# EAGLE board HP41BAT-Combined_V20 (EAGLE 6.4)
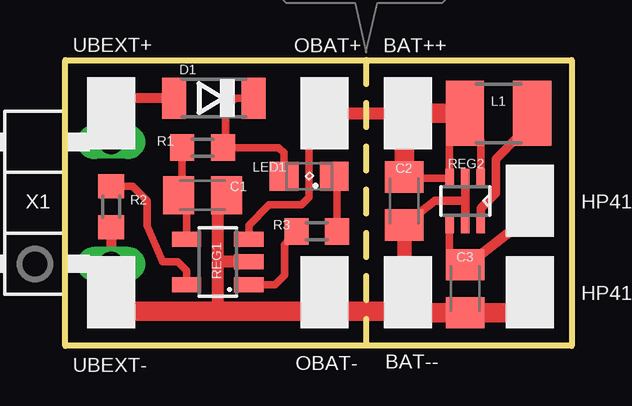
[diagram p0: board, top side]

Size 21.11 x 11.91 mm. Coordinates in mm from the lower left corner, seen from the top.
Outline: 21.11,0 0,0 0,11.91 21.11,11.91 21.11,0
Copper layers (1*16): Top 0.035mm / dielectric 1.5mm / Bottom 0.035mm
Design rules "pcb-pool-2009": minimum track width 6mil, minimum drill 12mil, track to track 6mil, track to pad 6mil, pad to pad 6mil, via to via 6mil, smd to smd 6mil, copper to edge 20mil, drill to drill 8mil, minimum pad ring 8mil, minimum via ring 6mil, stop-mask expansion 3mil, vias tented up to drill 0mil, thermal gap 8mil
Milling: 7 lines

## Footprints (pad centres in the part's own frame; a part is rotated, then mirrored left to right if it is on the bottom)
AKKI_LOETPAD_2X3_T = smd 2 x 3: P$1 0,0
C0805K = smd 1.3 x 1.6: 1 -1,0; 2 1,0
SOD80-R = smd 1 x 1.7: A 1.65,0; C -1.65,0
AKKI_LOETPAD_2X3_T_HOLE = smd 2 x 3: P$1 0,0 | hole 0.8: 0,0
R1210 = smd 1.6 x 2.7: 1 -1.4,0; 2 1.4,0
SML0805 = smd 1.2 x 1.2: A 1.05,0; C -1.05,0
R0603 = smd 1 x 1.1: 1 -0.85,0; 2 0.85,0
TSOT23-5 = smd 0.62 x 1.22: 1 -0.95,-1.3; 2 0,-1.3; 3 0.95,-1.3; 4 0.95,1.3; 5 -0.95,1.3
SC70-6 = smd 0.35 x 0.8: 1 -0.65,-0.95; 2 0,-0.95; 3 0.65,-0.95; 4 0.65,0.95; 5 0,0.95; 6 -0.65,0.95
1X03-1/90 = drill 1.016 long: 1 -2.54,-3.81; 3 2.54,-3.81

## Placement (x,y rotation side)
BAT++  AKKI_LOETPAD2X3_T  [AKKI_LOETPAD_2X3_T]  14.29,9.68 180 top
BAT--  AKKI_LOETPAD2X3_T  [AKKI_LOETPAD_2X3_T]  14.29,2.22 0 top
C1  2u2  [C0805K]  5.71,6.27 0 top
C2  2u2  [C0805K]  14.13,6.03 270 top
C3  22u  [C0805K]  16.67,2.38 270 top
D1  LL103  [SOD80-R]  6.19,10.32 180 top
HP41+  AKKI_LOETPAD2X3_T_HOLE  [AKKI_LOETPAD_2X3_T_HOLE]  19.37,6.03 180 top
HP41-  AKKI_LOETPAD2X3_T_HOLE  [AKKI_LOETPAD_2X3_T_HOLE]  19.37,2.22 180 top
L1  10u  [R1210]  18.06,9.68 0 top
LED1  red  [SML0805]  10.16,7.06 180 top
OBAT+  AKKI_LOETPAD2X3_T  [AKKI_LOETPAD_2X3_T]  10.79,9.68 0 top
OBAT-  AKKI_LOETPAD2X3_T  [AKKI_LOETPAD_2X3_T]  10.79,2.22 0 top
R1  4E7  [R0603]  5.71,8.26 0 top
R2  47k  [R0603]  1.91,5.79 90 top
R3  390E  [R0603]  10.48,4.76 0 top
REG1  LTC4054-4.2  [TSOT23-5]  6.35,3.49 90 top
REG2  LTC3525-5  [SC70-6]  16.67,6.03 180 top
UBEXT+  AKKI_LOETPAD2X3_T  [AKKI_LOETPAD_2X3_T]  1.91,9.68 0 top
UBEXT-  AKKI_LOETPAD2X3_T  [AKKI_LOETPAD_2X3_T]  1.91,2.22 0 top
X1  [1X03-1/90]  -1.91,5.95 90 top

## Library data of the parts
BAT++ BAT-- D1 HP41+ HP41- OBAT+ OBAT- REG1 REG2 UBEXT+ UBEXT- = Akki_V6
C1 = rcl; TEXH: X7R
C2 C3 = rcl; TECH: X7R
L1 = Akki_V6; MAT: LQH3C; SIZE: 1210
LED1 = led; SIZE: 0805
R1-R3 = Akki_V6; SIZE: 0603
X1 = AkkiTestV6

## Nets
GND: BAT--.P$1 C1.2 C2.2 C3.2 HP41-.P$1 OBAT-.P$1 R2.1 REG1.2 REG2.2 REG2.5 UBEXT-.P$1 X1.1
N$6: C1.1 R1.1 REG1.4
N$7: L1.2 REG2.6
N$8: C3.1 HP41+.P$1 REG2.4
N$12: R2.2 REG1.5
N$13: R3.1 REG1.1
N$14: D1.C LED1.A R1.2
N$15: LED1.C R3.2
N$16: D1.A UBEXT+.P$1 X1.3
VIN: BAT++.P$1 C2.1 L1.1 OBAT+.P$1 REG1.3 REG2.1 REG2.3

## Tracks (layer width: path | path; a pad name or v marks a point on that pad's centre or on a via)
GND
  Top 0.356: REG2.2 16.67,6.03 | 16.67,6.03 REG2.5 | C2.2 15.4,6.03 16.67,6.03
  Top 0.406: R2.1 X1.1 UBEXT-.P$1
  Top 0.457: C1.2 6.71,6.24
  Top 0.508: 6.71,6.24 6.71,6.16 6.35,5.79 6.35,3.49 | 6.35,3.49 6.35,1.43 | REG1.2 6.35,3.49
  Top 0.61: C2.2 14.13,2.54 14.45,2.22 BAT--.P$1
  Top 0.813: HP41-.P$1 18.53,1.38 C3.2 15.13,1.38 BAT--.P$1 14.29,1.43 10.79,1.43 10.79,1.59 | 10.79,1.59 OBAT-.P$1 | 10.79,1.59 10.48,1.59 10.32,1.43 6.35,1.43 2.38,1.43 1.91,1.91 UBEXT-.P$1
N$6
  Top 0.305: R1.1 4.87,6.42 C1.1 5.05,5.94 REG1.4
N$7
  Top 0.356: REG2.6 17.32,5.73 17.94,6.35 17.94,7.78 18.89,8.73 18.89,9.12 L1.2
N$8
  Top 0.305: REG2.4 16.02,3.83 16.19,3.65 16.4,3.65 C3.1
  Top 0.406: HP41+.P$1 19.37,5.56 18.57,4.76 17.14,3.65 C3.1
N$12
  Top 0.305: REG1.5 5.05,3.13 4.68,3.49 4.05,3.49 3.41,5 3.41,6.03 2.8,6.64 R2.2
N$13
  Top 0.305: REG1.1 8.73,2.54 9.13,2.94 9.13,4.21 9.29,4.37 9.29,4.42 R3.1
N$14
  Top 0.305: D1.C 7.06,10.32 6.67,9.92 6.67,8.42 R1.2 8.89,8.26 9.11,8.04 LED1.A
N$15
  Top 0.305: R3.2 11.33,6.95 LED1.C
N$16
  Top 0.406: D1.A 2.54,10.32 UBEXT+.P$1 X1.3
VIN
  Top 0.305: C2.1 14.5,6.98 REG2.3 16.02,8.56 16.19,8.73 17.14,8.73 17.32,8.56 REG2.1 | REG1.3 7.65,5.03 8.49,5.87 9.84,5.87 10.16,6.19 10.16,9.05 OBAT+.P$1
  Top 0.457: 13.81,8.41 14.13,8.73
  Top 0.508: OBAT+.P$1 BAT++.P$1
  Top 0.813: C2.1 14.13,8.73 14.13,9.21 14.45,9.53 BAT++.P$1 L1.1

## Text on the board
tDocu: CARVE BOTTOM! | UBEXT+ | X1 is optional | UBEXT- | HP41BAT-COMBINED V2.0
